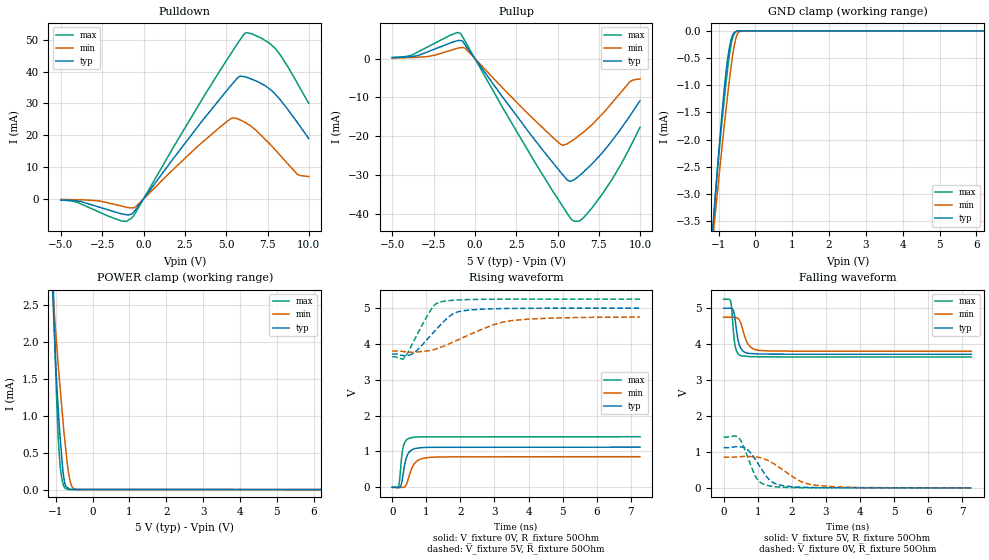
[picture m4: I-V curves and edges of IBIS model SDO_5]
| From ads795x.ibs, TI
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|   3-state SDO model 5V
[Model]   SDO_5
Model_type   3-state
|Signals   SDO
Vmeas = 2.5
Vref = 2.5
Cref = 15pF
Rref = 50
| variable   typ   min   max
|C_comp Output in tri-state
C_comp   7.9747161e-13   9.4032303e-13   6.5714514e-13
|C_comp Output High
|C_comp   1.9431567e-10   1.0014936e-10   3.2697328e-10
|C_comp Output Low
|C_comp   1.1328731e-10   6.1394150e-11   2.0665026e-10
[Voltage Range]   5   4.75   5.25
[Temperature Range]   27   125   -40
[Pullup Reference]   5   4.75   5.25
[Pulldown Reference]   0   -0   0
[Power Clamp Reference]   5   4.75   5.25
[GND Clamp Reference]   0   0   0
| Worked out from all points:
|   slope of the pulldown table from 0 to 0.75 V, typ, clamps not added: 142 ohm
|   slope of the pullup table from 0 to 0.75 V, typ, clamps not added: 168 ohm
|   GND clamp passes 1 mA (typ) near -0.83 V on its own axis
|   POWER clamp passes 1 mA (typ) near -0.92 V on its own axis
|   falling waveform, V_fixture 5V, R_fixture 50Ohm: 20-80 % time 136ps typ, 212ps min, 94.5ps max; typ from 5 V to 3.72 V
|   rising waveform, V_fixture 0V, R_fixture 50Ohm: 20-80 % time 146ps typ, 223ps min, 99.7ps max; typ from 0 V to 1.12 V
|   rising waveform, V_fixture 5V, R_fixture 50Ohm: 20-80 % time 763ps typ, 1.42ns min, 547ps max; typ from 3.72 V to 5 V
|   falling waveform, V_fixture 0V, R_fixture 50Ohm: 20-80 % time 486ps typ, 831ps min, 364ps max; typ from 1.12 V to 0 V
[Pulldown]
|   Voltage   I(typ)   I(min)   I(max)
-5V       -320uA     -173.3uA   -370.5uA
-4.04V    -652.7uA   -265.5uA   -1.002mA
-1.311V   -4.716mA   -2.274mA   -6.98mA
-707.2mV  -4.748mA   -2.847mA   -5.983mA
-464.2mV  -3.261mA   -2.424mA   -4.158mA
5.249V    35.37mA    25.1mA     45.34mA
5.83V     38.57mA    24.83mA    49.91mA
6.182V    38.28mA    23.91mA    52.21mA
7.163V    36.1mA     19.71mA    50.37mA
7.977V    32.81mA    15.33mA    47.18mA
9.293V    24.06mA    7.751mA    36.41mA
9.985V    18.99mA    7.033mA    30.03mA
[GND Clamp]
|   Voltage   I(typ)   I(min)   I(max)
-5V       -39.42mA   -31.32mA   -49.69mA
-1.155V   -3.607mA   -3.811mA   -3.717mA
-1.104V   -3.154mA   -3.461mA   -3.213mA
-1.022V   -2.463mA   -2.909mA   -2.507mA
-925.1mV  -1.675mA   -2.268mA   -1.791mA
-775.8mV  -640.2uA   -1.317mA   -828.6uA
-712.7mV  -338.3uA   -948.4uA   -484.2uA
-639mV    -119.5uA   -557.4uA   -187.2uA
-568.3mV  -29.29uA   -250.4uA   -48.99uA
-508.8mV  -6.751uA   -89.06uA   -9.397uA
-296.2mV  -586nA     -279.1nA   -624.8nA
9.985V    0A         0A         0A
[Pullup]
|   Voltage   I(typ)   I(min)   I(max)
-5V       232.9uA    156.6uA    284.4uA
-3.846V   502uA      261.7uA    832.6uA
-893.2mV  4.656mA    2.781mA    6.575mA
-551.9mV  3.3mA      2.524mA    4.166mA
1.721V    -10.18mA   -7.773mA   -12.97mA
5.175V    -29.27mA   -22.09mA   -37.25mA
5.739V    -31.7mA    -21.56mA   -40.89mA
6.012V    -31.25mA   -20.81mA   -41.96mA
6.525V    -29.45mA   -19.13mA   -41.27mA
7.724V    -24.2mA    -14.21mA   -34.85mA
9.381V    -14.74mA   -5.945mA   -22.93mA
9.985V    -10.87mA   -5.255mA   -17.75mA
[POWER Clamp]
|   Voltage   I(typ)   I(min)   I(max)
-5V       75.77mA    59.83mA    93.41mA
-1.078V   2.582mA    2.669mA    2.93mA
-1.05V    2.244mA    2.455mA    2.422mA
-972.8mV  1.407mA    1.944mA    1.164mA
-914.8mV  940.7uA    1.564mA    537.8uA
-836.5mV  424.2uA    1.107mA    150.1uA
-796.8mV  213.4uA    876.1uA    66.2uA
-744.6mV  67.29uA    616.9uA    15.71uA
-620.5mV  6.412uA    131.7uA    1.083uA
-568.3mV  933.5nA    43.8uA     1.077uA
-436.2mV  921.8nA    1.216uA    1.064uA
9.985V    0A         0A         0A
[Ramp]
R_load = 50
|   typ   min   max
dV/dt_r   0.672068/1.4606e-010   0.512528/2.19104e-010  0.846698/9.93401e-011
dV/dt_f   0.768928/1.3559e-010   0.568592/2.11904e-010  0.963984/9.4168e-011
[Falling Waveform]
V_fixture = 5V
V_fixture_min = 4.75V
V_fixture_max = 5.25V
R_fixture = 50Ohm
C_fixture = 0F
|   Time   V(typ)   V(min)   V(max)
0s        5V         4.75V      5.25V
208.1ps   5.002V     4.75V      5.196V
239.3ps   4.99V      4.75V      4.976V
293.6ps   4.922V     4.75V      4.31V
341.8ps   4.665V     4.748V     3.944V
434.7ps   4.079V     4.707V     3.727V
530.8ps   3.853V     4.508V     3.675V
727.8ps   3.746V     3.989V     3.658V
1.057ns   3.728V     3.825V     3.651V
7.268ns   3.718V     3.802V     3.643V
[Rising Waveform]
V_fixture = 0V
V_fixture_min = 0V
V_fixture_max = 0V
R_fixture = 50Ohm
C_fixture = 0F
|   Time   V(typ)   V(min)   V(max)
0s        -168.2nV   -234.4nV   -190.9nV
186.6ps   -7.384mV   -2.114mV   29.09mV
216.8ps   -1.302mV   -2.457mV   201.1mV
265.1ps   70.45mV    -3.004mV   719mV
326.7ps   406.1mV    1.617mV    1.138V
404ps     793.5mV    57.62mV    1.307V
541.3ps   1.023V     445.4mV    1.381V
795ps     1.099V     773mV      1.405V
1.253ns   1.117V     843.3mV    1.408V
7.268ns   1.12V      854.2mV    1.411V
[Rising Waveform]
V_fixture = 5V
V_fixture_min = 4.75V
V_fixture_max = 5.25V
R_fixture = 50Ohm
C_fixture = 0F
|   Time   V(typ)   V(min)   V(max)
0s        3.718V     3.802V     3.643V
370.5ps   3.667V     3.783V     3.621V
693.8ps   3.791V     3.77V      4.19V
1.134ns   4.24V      3.822V     4.954V
1.439ns   4.554V     3.913V     5.177V
1.73ns    4.807V     4.029V     5.214V
2.023ns   4.915V     4.154V     5.231V
2.911ns   4.98V      4.513V     5.246V
3.492ns   4.99V      4.649V     5.248V
7.268ns   5V         4.75V      5.25V
[Falling Waveform]
|Gnd
V_fixture = 0V
V_fixture_min = 0V
V_fixture_max = 0V
R_fixture = 50Ohm
C_fixture = 0F
|   Time   V(typ)   V(min)   V(max)
0s        1.12V      854.2mV    1.411V
449.2ps   1.147V     865.4mV    1.393V
666.2ps   1.092V     878.3mV    961.8mV
966.6ps   741.9mV    859.6mV    271.7mV
1.104ns   538.8mV    832.9mV    135.1mV
1.332ns   236mV      747.3mV    56.46mV
1.611ns   87.63mV    584.9mV    23.77mV
2.243ns   19.05mV    188.8mV    3.553mV
2.731ns   6.623mV    69.49mV    2.747mV
7.268ns   -168.2nV   -234.4nV   -190.9nV
